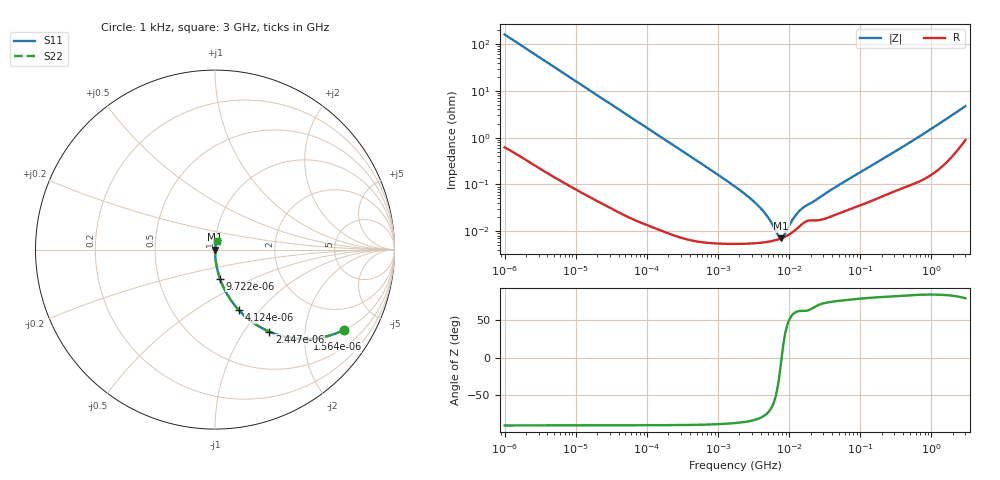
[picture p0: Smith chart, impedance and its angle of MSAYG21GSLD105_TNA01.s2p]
! MSAYG21GSLD105_TNA01  S-PARAMETER MODEL  ( Standard Model )
! Model Generated by TAIYO YUDEN Corporation (http://www.ty-top.com)
! Version 1.0
! TAIYO YUDEN Control No. 220601
! Copyright(c) 2012 TAIYO YUDEN CO.,LTD. All Rights Reserved.
! Product Description (link to TY-COMPAS)
! https://ds.yuden.co.jp/TYCOMPAS/or/detail?pn=MSAYG21GSLD105KTNA01&u=M
! Products Name : Multilayer Ceramic Capacitors
! Characteristics :
!  Capacitance : 1 [uF] , Rated Voltage : 35 [V] , TCC : X5R
!  Case Size : 2.0 x 1.25 / 0.079 x 0.049 [mm/inch] , Thickness : 1.25 / 0.049 [mm/inch]
!  (Conditions: Temperature = 25 [degC] , DC Bias Voltage = 0 [V])
! External Node Assignments :
!  1  o---| |---o  2
! GND o---------o GND
! Frequency Range : 1kHz  -  3GHz  [ 401 STEP ]
# MHZ S RI R 50
! Freq[MHz].  S11 Real  S11 Imag  S21 Real  S21 Imag  S12 Real  S12 Imag  S22 Real  S22 Imag
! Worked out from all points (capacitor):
!   401 points, 1 kHz to 3 GHz, reference 50 ohm
!   read as one part in series: C = 992 nF near 1.077 kHz
!   lowest |Z| = 7.05 mohm at 7.696 MHz (marker M1)
!   series resonance near 7.824 MHz, so ESL is about 420 pH
!   S11 on the Smith chart (normalised r, x): 1 kHz: 1.01, -3.20; 1.564 kHz: 1.01, -2.05; 2.447 kHz: 1.01, -1.31; 4.124 kHz: 1.00, -0.78; 9.722 kHz: 1.00, -0.33; 3 GHz: 1.02, +0.09
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0.001  0.719 -0.4476  0.281 0.4476  0.281 0.4476  0.719 -0.4476
0.001564  0.5126 -0.4978  0.4874 0.4978  0.4874 0.4978  0.5126 -0.4978
0.002447  0.302 -0.457  0.698 0.457  0.698 0.457  0.302 -0.457
0.004124  0.1331 -0.3376  0.8669 0.3376  0.8669 0.3376  0.1331 -0.3376
0.005988  0.0684 -0.2502  0.9316 0.2502  0.9316 0.2502  0.0684 -0.2502
0.009722  0.0275 -0.1612  0.9725 0.1612  0.9725 0.1612  0.0275 -0.1612
0.01216  0.0179 -0.1302  0.9821 0.1302  0.9821 0.1302  0.0179 -0.1302
0.033275  0.00265 -0.0485  0.9973 0.0485  0.9973 0.0485  0.00265 -0.0485
0.147855  0.000228 -0.011  0.9998 0.011  0.9998 0.011  0.000228 -0.011
1.732051  5.42e-05 -0.000897  0.9999 0.000897  0.9999 0.000897  5.42e-05 -0.000897
2.812335  5.46e-05 -0.000506  0.9999 0.000506  0.9999 0.000506  5.46e-05 -0.000506
3.93371  5.65e-05 -0.00031  0.9999 0.00031  0.9999 0.00031  5.65e-05 -0.00031
4.919932  5.9e-05 -0.000201  0.9999 0.000201  0.9999 0.000201  5.9e-05 -0.000201
6.629817  6.51e-05 -6.93e-05  0.9999 6.93e-05  0.9999 6.93e-05  6.51e-05 -6.93e-05
7.696136  7.02e-05 -6.77e-06  0.9999 6.77e-06  0.9999 6.77e-06  7.02e-05 -6.77e-06
8.933959  7.75e-05 5.53e-05  0.9999 -5.53e-05  0.9999 -5.53e-05  7.75e-05 5.53e-05
12.03889  0.000104 0.000181  0.9999 -0.000181  0.9999 -0.000181  0.000104 0.000181
13.97519  0.000127 0.000241  0.9999 -0.000241  0.9999 -0.000241  0.000127 0.000241
21.06097  0.000171 0.000376  0.9998 -0.000376  0.9998 -0.000376  0.000171 0.000376
44.39505  0.000225 0.00084  0.9998 -0.00084  0.9998 -0.00084  0.000225 0.00084
256.0921  0.000659 0.00422  0.9993 -0.00422  0.9993 -0.00422  0.000659 0.00422
3000  0.0109 0.0454  0.9891 -0.0454  0.9891 -0.0454  0.0109 0.0454
